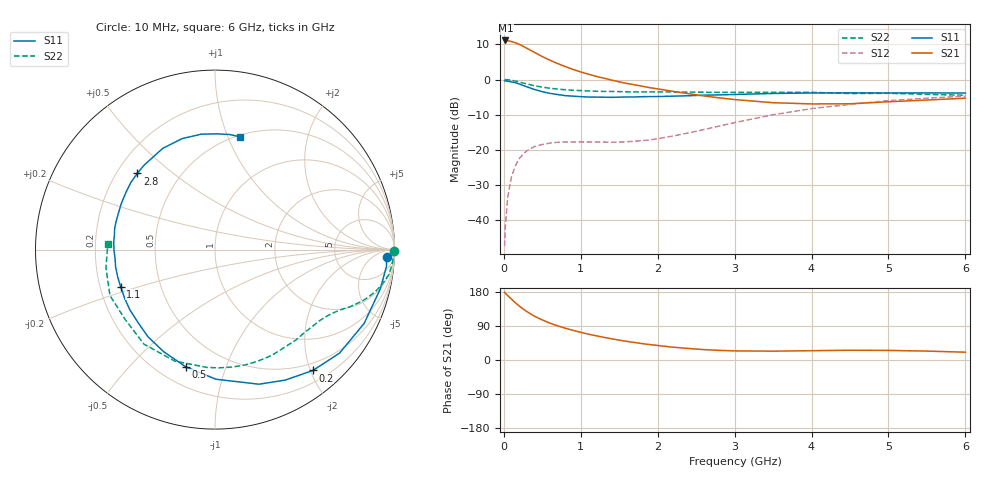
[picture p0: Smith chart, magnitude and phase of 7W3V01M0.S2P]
! Infineon Technologies  Discrete & RF Semiconductors
! BFS17W
! Si NPN RF Bipolar Junction Transistor in SOT323
! VCE = 3 V  IC = 1 mA
! Common Emitter S-Parameters:  August  1999
# GHz  S  MA  R  50
!  f  S11  S21  S12  S22
! GHz  MAG  ANG  MAG  ANG  MAG  ANG  MAG  ANG
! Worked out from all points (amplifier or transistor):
!   36 points, 10 MHz to 6 GHz, reference 50 ohm
!   highest |S21| = 11.1 dB at 20 MHz (marker M1)
!   |S21| within 3 dB of that: start of sweep to 365.7 MHz
!   unconditionally stable (mu >= 1): 1.032 GHz to end of sweep
!   at 250 MHz: K = 0.26, MSG = 15.3 dB, |S12| = -21.2 dB
!   at 1.4 GHz: K = 1.28, MAG = 5.6 dB, |S12| = -17.8 dB
!   at 6 GHz: K = 1.10, MAG = -2.2 dB, |S12| = -4.7 dB
!   S11 on the Smith chart (normalised r, x): 10 MHz: 23, -23; 200 MHz: 0.38, -2.04; 500 MHz: 0.31, -0.73; 1.1 GHz: 0.29, -0.17; 2.8 GHz: 0.28, +0.38; 6 GHz: 0.52, +1.11
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0.01  0.9569 -2.5  3.59 178.8  0.0043 88.3  0.9999 -0.3
0.02  0.9598 -5.6  3.594 176.2  0.0082 84.4  0.9967 -1.7
0.05  0.9466 -13.4  3.574 169.9  0.0213 83.1  0.9917 -4.1
0.1  0.9272 -26.3  3.46 160.6  0.0421 74.9  0.9794 -8.1
0.15  0.9024 -39.7  3.331 150.9  0.0597 67.1  0.9514 -11.7
0.2  0.8667 -51.0  3.167 142.5  0.0751 61.5  0.9237 -14.7
0.25  0.8253 -61.8  2.968 134.7  0.087 55.6  0.8932 -17.3
0.3  0.789 -71.9  2.776 127.7  0.0976 51.3  0.8671 -19.4
0.4  0.7222 -89.6  2.431 115.4  0.112 43.7  0.8174 -22.9
0.5  0.673 -104.1  2.122 105.7  0.1197 38.3  0.7804 -25.3
0.6  0.6366 -116.7  1.882 97.2  0.1252 34.9  0.7527 -27.6
0.7  0.6129 -127.5  1.687 90.1  0.1287 32.7  0.7322 -29.8
0.9  0.5811 -144.7  1.393 78.2  0.1297 30.2  0.7046 -34.2
1.1  0.5648 -158.6  1.192 68.1  0.1302 30.4  0.6895 -38.9
1.6  0.5658 175.9  0.88 49.1  0.1309 38.5  0.67 -52.0
2.2  0.5813 154.2  0.68 33.8  0.1578 54.2  0.6658 -69.5
2.8  0.606 135.6  0.55 25.4  0.2184 61.7  0.6592 -88.1
3.5  0.6348 117.3  0.469 23.3  0.3164 60.2  0.6605 -109.9
4  0.6449 106.5  0.451 24.6  0.387 54.6  0.6587 -127.0
4.5  0.6476 96.8  0.453 25.7  0.4434 48.1  0.6337 -142.6
5.5  0.6465 82.7  0.512 23.5  0.5438 35.1  0.6158 -170.6
6  0.6433 77.5  0.544 20.6  0.5822 29.0  0.598 177.1
